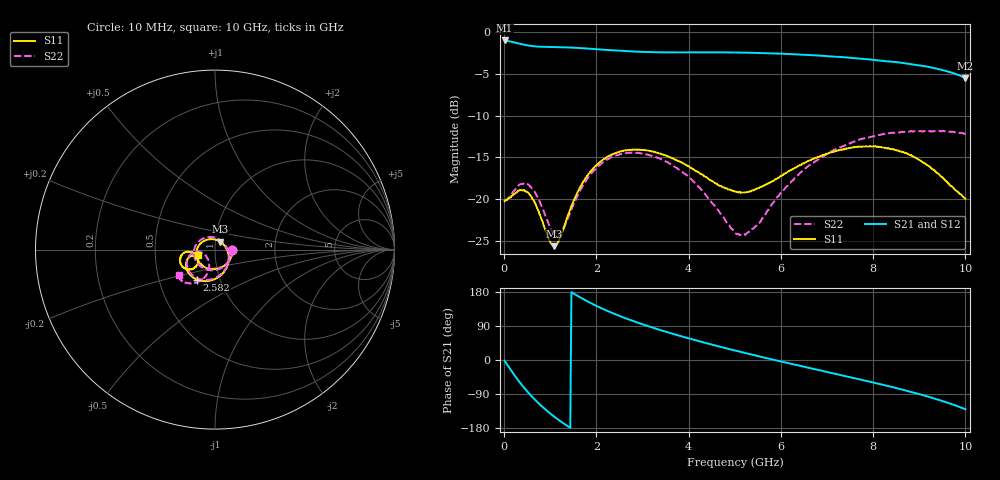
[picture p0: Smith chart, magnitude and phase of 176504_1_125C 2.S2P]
!  2-Port S-parameters saved by WinCal
! VAR MeasName=S-Parameters (CALIBRATED_DATA) read from VNA (N5242A)
! VAR MeasDate=2017-11-2 17:34:18
! VAR NAME=176504_1_125C 2
! VAR FILENAME=176504_1_125C 2.S2P
! VAR DATE=2017-11-2 17:34:18
! VAR PHYS_PORTS=2,3
# Hz S DB R 50
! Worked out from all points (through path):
!   401 points, 10 MHz to 10 GHz, reference 50 ohm
!   highest |S21| = -1.02 dB at 10 MHz (marker M1); lowest = -5.5 dB at 10 GHz (marker M2)
!   lowest |S11| = -25.6 dB at 1.084 GHz (marker M3), VSWR 1.11, Z = 52.6 + j4.71 ohm
!   |S11| at or under -10 dB: start of sweep to end of sweep
!   |S22| runs from -24.5 to -11.8 dB; largest |S21 - S12| = 0.013
!   S11 on the Smith chart (normalised r, x): 10 MHz: 1.22, -0.01; 2.582 GHz: 0.78, -0.27; 10 GHz: 0.82, -0.05
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1e7  -20.22 -2.6  -1.02 -2.2  -1.02 -2.2  -20.22 -2.3
1.34875e8  -19.81 -52.2  -1.15 -24.7  -1.15 -24.7  -19.64 -55.1
2.5975e8  -19.21 -93.5  -1.31 -46.2  -1.32 -46.2  -18.70 -96.9
4.5955e8  -19.06 -145.3  -1.57 -77.1  -1.57 -77.0  -18.18 -148.4
7.34275e8  -21.27 155.2  -1.75 -112.7  -1.75 -112.7  -19.87 154.0
9.091e8  -23.93 113.6  -1.78 -132.1  -1.79 -132.0  -22.19 116.3
1.083925e9  -25.61 58.3  -1.81 -149.4  -1.80 -149.3  -24.25 68.3
1.2088e9  -24.66 19.4  -1.82 -160.7  -1.82 -160.6  -24.21 30.5
1.35865e9  -22.35 -15.5  -1.85 -173.2  -1.85 -173.2  -22.61 -7.5
1.683325e9  -18.23 -59.9  -1.94 162.8  -1.94 162.9  -18.63 -57.4
2.1079e9  -15.42 -94.4  -2.11 136.7  -2.10 136.7  -15.73 -94.4
2.582425e9  -14.22 -120.5  -2.28 112.4  -2.28 112.6  -14.56 -122.4
3.35665e9  -14.51 -148.5  -2.44 80.1  -2.46 80.3  -15.10 -153.3
4.230775e9  -16.85 -164.3  -2.44 49.4  -2.43 49.9  -18.59 -172.6
5.005e9  -19.08 -157.2  -2.46 25.0  -2.46 25.4  -23.91 -156.1
5.379625e9  -18.94 -147.3  -2.50 13.9  -2.50 14.2  -23.53 -127.9
6.05395e9  -17.06 -138.3  -2.62 -5.4  -2.63 -5.0  -18.91 -107.0
6.678325e9  -15.20 -140.7  -2.78 -22.7  -2.80 -22.3  -15.69 -110.0
7.577425e9  -13.80 -151.6  -3.14 -47.5  -3.16 -47.1  -13.11 -122.4
8.35165e9  -13.97 -165.1  -3.53 -69.5  -3.58 -69.1  -12.11 -132.2
9.225775e9  -16.11 -175.3  -4.21 -98.1  -4.24 -97.2  -11.84 -139.6
1e10  -19.93 -163.3  -5.52 -129.9  -5.53 -129.0  -12.18 -145.2
